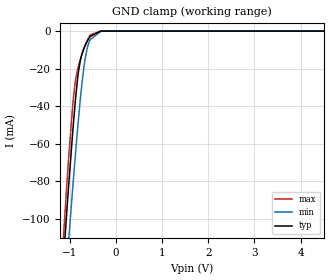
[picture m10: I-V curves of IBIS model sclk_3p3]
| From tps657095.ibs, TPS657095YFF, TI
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|   sclk_3p3 Model
[Model]   sclk_3p3
Model_type   Input
Vinl = 0.4
Vinh = 1.2
|   typ   min   max
|   (nom PVT)   (fast PVT)   (slow PVT)
C_comp   3.211e-12   3.166e-12   3.402e-12
| Where nom  PVT is Nominal Process, 3.3V, 27C
|   Fast PVT is Strong Process,  3.6V, -40C
|   Slow PVT is Weak Process,   3V, 125C
[Voltage Range]   3.3   3   3.6
|Junction Temperature
[Temperature Range]   27   125   -40
[Power Clamp Reference]   3.3   3   3.6
[GND Clamp Reference]   0   0   0
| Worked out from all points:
|   GND clamp passes 1 mA (typ) near -0.41 V on its own axis
[GND Clamp]
|   Voltage   I(typ)   I(min)   I(max)
-3.3V     -1.008A    -964.3mA   -1.067A
-1.201V   -145.4mA   -171.2mA   -134.7mA
-1.046V   -90.4mA    -119.4mA   -75.93mA
-1.023V   -82.44mA   -111.8mA   -67.63mA
-927.3mV  -51.53mA   -81.41mA   -37.5mA
-873.6mV  -36.14mA   -65.15mA   -26.19mA
-808.8mV  -21.47mA   -46.63mA   -18.55mA
-735mV    -12.24mA   -27.96mA   -12.41mA
-672mV    -8.096mA   -15.63mA   -7.973mA
-552mV    -2.772mA   -4.461mA   -1.979mA
-240mV    -2.402uA   -29.4uA    -383.3nA
6.6V      0A         0A         0A
[POWER Clamp]
|   Voltage   I(typ)   I(min)   I(max)
-3.3V     0A         0A         0A
0V        0A         0A         0A
6.6V      0A         0A         0A
